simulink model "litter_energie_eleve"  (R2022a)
settings: Solver=ode14x  StartTime=0.0  StopTime=560  FixedStep=0.001  RelTol=1e-4  EnableMultiTasking=on
libraries: fl_lib x26, nesl_utility x12, ee_lib x2, simulink x1

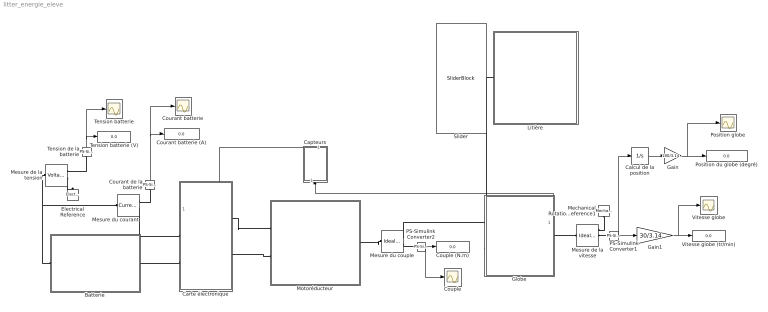
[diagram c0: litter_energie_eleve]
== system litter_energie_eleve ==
  Batterie : Subsystem
  Calcul de la position : Integrator
  Capteurs : Subsystem
  Carte électronique : Subsystem
  Couple : Scope
  Couple (N.m) : Display
  Courant batterie : Scope
  Courant batterie (A) : Display
  Courant de la batterie : nesl_utility/PS-Simulink Converter  PhysicalDomain=network_engine_domain  SubClassName=ps_output  LeftPortType=input  RightPortType=output  PseudoPeriodic=off  Frequencies=[]  VectorFormat=1-D array  Unit=inherit  AffineConversion=off
  Electrical Reference : fl_lib/Electrical/Electrical Elements/Electrical Reference
  Gain : Gain  Gain=180/3.14
  Gain1 : Gain  Gain=30/3.14
  Globe : Subsystem
  Litière : Subsystem
  Mechanical Rotational Reference1 : fl_lib/Mechanical/Rotational Elements/Mechanical Rotational Reference
  Mesure de la tension : fl_lib/Electrical/Electrical Sensors/Voltage Sensor
  Mesure de la vitesse : fl_lib/Mechanical/Mechanical Sensors/Ideal Rotational Motion Sensor  wrap_angle=simscape.enum.onoff.off  offset=0 rad
  Mesure du couple : fl_lib/Mechanical/Mechanical Sensors/Ideal Torque Sensor
  Mesure du courant : fl_lib/Electrical/Electrical Sensors/Current Sensor
  Motoréducteur : Subsystem
  PS-Simulink Converter1 : nesl_utility/PS-Simulink Converter  PhysicalDomain=network_engine_domain  SubClassName=ps_output  LeftPortType=input  RightPortType=output  PseudoPeriodic=off  Frequencies=[]  VectorFormat=1-D array  Unit=inherit  AffineConversion=off
  PS-Simulink Converter2 : nesl_utility/PS-Simulink Converter  PhysicalDomain=network_engine_domain  SubClassName=ps_output  LeftPortType=input  RightPortType=output  PseudoPeriodic=off  Frequencies=[]  VectorFormat=1-D array  Unit=inherit  AffineConversion=off
  Position du globe (degré) : Display
  Position globe : Scope
  Slider : SliderBlock  ScaleMax=4.5
  Tension batterie : Scope
  Tension batterie (V) : Display
  Tension de la batterie : nesl_utility/PS-Simulink Converter  PhysicalDomain=network_engine_domain  SubClassName=ps_output  LeftPortType=input  RightPortType=output  PseudoPeriodic=off  Frequencies=[]  VectorFormat=1-D array  Unit=inherit  AffineConversion=off
  Vitesse globe : Scope
  Vitesse globe (tr/min) : Display
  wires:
  Courant de la batterie/1 -> Courant batterie/1, Courant batterie (A)/1
  Tension de la batterie/1 -> Tension batterie/1, Tension batterie (V)/1
  Calcul de la position/1 -> Gain/1
  PS-Simulink Converter1/1 -> Calcul de la position/1, Gain1/1
  PS-Simulink Converter2/1 -> Couple/1, Couple (N.m)/1
  Globe/1(Out1) -> Capteurs/1(In1)
  Capteurs/1(Out1) -> Carte électronique/1(angle)
  Gain/1 -> Position globe/1, Position du globe (degré)/1
  Gain1/1 -> Vitesse globe/1, Vitesse globe (tr/min)/1
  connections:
  Courant de la batterie/LConn1 -- Mesure du courant/RConn1
  PS-Simulink Converter1/LConn1 -- Mesure de la vitesse/RConn2
  Mechanical Rotational Reference1/LConn1 -- Mesure de la vitesse/RConn1
  Tension de la batterie/LConn1 -- Mesure de la tension/RConn1
  Mesure de la tension/LConn1 -- Batterie/LConn1 -- Mesure du courant/LConn1
  Mesure de la tension/RConn2 -- Electrical Reference/LConn1
  Mesure du courant/RConn2 -- Carte électronique/LConn1
  Batterie/RConn1 -- Carte électronique/LConn2
  Carte électronique/RConn1 -- Motoréducteur/LConn1
  Carte électronique/RConn2 -- Motoréducteur/LConn2
  Mesure du couple/LConn1 -- Motoréducteur/RConn1
  Globe/RConn1 -- Mesure de la vitesse/LConn1
  Mesure du couple/RConn2 -- PS-Simulink Converter2/LConn1
  Mesure du couple/RConn1 -- Globe/LConn1
  Globe/LConn2 -- Litière/RConn1

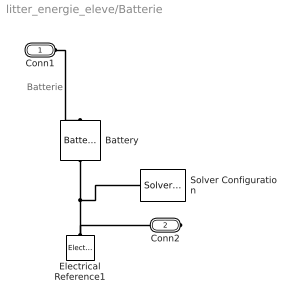
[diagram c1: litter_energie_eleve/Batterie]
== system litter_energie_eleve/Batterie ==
  note: Batterie
  Battery : ee_lib/Sources/Battery  Vnom=12 V  prm_dir=ee.enum.batterybasic.prm_dir.disabled  R1_dis=2 Ohm  R1_ch=2 Ohm  R1=2 Ohm  prm_AH=ee.enum.batterybasic.prm_AH.infinite  AH=50 A*hr  V1=11.5 V  AH1=25 A*hr  prm_R2=ee.enum.batterybasic.prm_R2.disabled  R2=2000 Ohm  prm_dyn=ee.enum.batterybasic.prm_dyn.off  Rp1=0.005 Ohm  tau1=30 s  Rp2=0.005 Ohm  tau2=30 s  Rp3=0.005 Ohm  tau3=30 s  Rp4=0.005 Ohm  tau4=30 s  Rp5=0.005 Ohm  tau5=30 s  prm_fade=ee.enum.batterybasic.prm_fade.disabled  N_fade=100  AH_fade=45 A*hr  R1_fade=2.02 Ohm  R1_ch_fade=2.02 Ohm  V1_fade=10.35 V  prm_age=ee.enum.batterybasic.prm_age.disabled  prm_age_OCV=ee.enum.batterybasic.prm_age_OCV.OCV  OCV_age=0.9  SOC_age=60  delta_time_age_vec=[0] d  temperature_age_vec=[273] K  OCV_scaling_age=2.2134e6  OCV_offset_age=1.632e6  temp_exp_age=0.515833569 V  t_exp_age=0.75  i_specify=off  i_priority=None  i=0 A  i_nominal_specify=off  i_nominal_unit=A  i_nominal_value=1  v_specify=off  v_priority=None  v=0 V  v_nominal_specify=off  v_nominal_unit=V  v_nominal_value=1  charge_specify=on  charge_priority=High  charge=13 A*hr  charge_nominal_specify=off  charge_nominal_unit=A*hr  charge_nominal_value=1  num_cycles_specify=off  num_cycles_priority=High  num_cycles=0  num_cycles_nominal_specify=off  num_cycles_nominal_unit=1  num_cycles_nominal_value=1  Tmeas=298.15 K  Tmeas_age=298.15 K  Vnom_T2=12 V  R1_T2=2.2 Ohm  R1_T2_dis=2.2 Ohm  R1_T2_ch=2.2 Ohm  V1_T2=11.4 V  R2_T2=2200 Ohm  Rp1_T2=0.005 Ohm  tau1_T2=30 s  Rp2_T2=0.005 Ohm  tau2_T2=30 s  Rp3_T2=0.005 Ohm  tau3_T2=30 s  Rp4_T2=0.005 Ohm  tau4_T2=30 s  Rp5_T2=0.005 Ohm  tau5_T2=30 s  Tmeas2=273.15 K  thermal_mass=30000 J/K  temperature_specify=off  temperature_priority=High  temperature=298.15 K  temperature_nominal_specify=off  temperature_nominal_unit=K  temperature_nominal_value=1
  Electrical Reference1 : fl_lib/Electrical/Electrical Elements/Electrical Reference
  Solver Configuration : nesl_utility/Solver Configuration  PhysicalDomain=network_engine_domain  SubClassName=solver  LeftPortType=input  RightPortType=generic  Tones=[]  Harmonics=[]  SimulateNoise=off  Profile=off  UseLocalSampling=off  EnableSwitchedLinearOptims=on  FrequencyDomain=off  UseCCode=off  RelTol=0.001  AbsTol=1e-06  MinStep=1e-09  ToWorkspace=off  RevertToSquareIcSolve=off  NumHomotopyIterations=100  PhasorMode=off  PhasorModeNumHarmonics=1  IndexReductionMethod=DerivativeReplacement  DoDC=off  ResidualTolerance=1e-4  UseLocalSolver=on  LocalSolverChoice=NE_TRAPEZOIDAL_ADVANCER  LocalSolverSampleTime=.001  DoFixedCost=on  MaxNonlinIter=3  MaxModeIter=2  ComputeImpulses=off  ImpulseIterations=2  LinearAlgebra=Sparse  LinearAlgebraNumThread=0  EquationFormulation=NE_TIME_EF  DelaysMemoryBudget=4096  AutomaticFiltering=on  FilteringTimeConstant=0.001  PartitionStorageMethod=AS_NEEDED  PartitionMemoryBudget=1024  PartitionMethod=FAST
  Conn1 : PMIOPort  Side=Left
  Conn2 : PMIOPort  Port=2  Side=Right
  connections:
  Electrical Reference1/LConn1 -- Conn2/RConn1 -- Battery/RConn1 -- Solver Configuration/RConn1
  Conn1/RConn1 -- Battery/LConn1

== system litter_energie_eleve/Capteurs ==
  In1 : Inport
  Integrator : Integrator
  Out1 : Outport
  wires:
  Integrator/1 -> Out1/1
  In1/1 -> Integrator/1

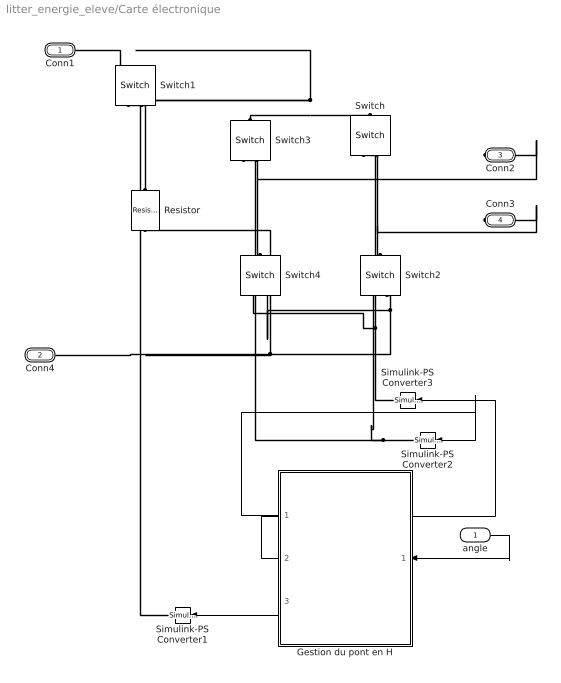
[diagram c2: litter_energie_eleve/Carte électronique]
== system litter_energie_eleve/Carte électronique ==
  angle : Inport
  Gestion du pont en H : Stateflow chart  TreatAsAtomicUnit=on
  Resistor : fl_lib/Electrical/Electrical Elements/Resistor  R=150 Ohm  i_specify=off  i_priority=None  i=0 A  i_nominal_specify=off  i_nominal_unit=A  i_nominal_value=1  v_specify=off  v_priority=None  v=0 V  v_nominal_specify=off  v_nominal_unit=V  v_nominal_value=1
  Simulink-PS Converter1 : nesl_utility/Simulink-PS Converter  PhysicalDomain=network_engine_domain  SubClassName=ps_input  LeftPortType=input  RightPortType=output  PseudoPeriodic=off  Frequencies=[]  NoiseDistribution=none  NoiseParameters=[]  Unit=1  AffineConversion=off  FilteringAndDerivatives=provide  SimscapeFilterOrder=1  InputFilterTimeConstant=0.001  UdotUserProvided=0
  Simulink-PS Converter2 : nesl_utility/Simulink-PS Converter  PhysicalDomain=network_engine_domain  SubClassName=ps_input  LeftPortType=input  RightPortType=output  PseudoPeriodic=off  Frequencies=[]  NoiseDistribution=none  NoiseParameters=[]  Unit=1  AffineConversion=off  FilteringAndDerivatives=provide  SimscapeFilterOrder=1  InputFilterTimeConstant=0.001  UdotUserProvided=0
  Simulink-PS Converter3 : nesl_utility/Simulink-PS Converter  PhysicalDomain=network_engine_domain  SubClassName=ps_input  LeftPortType=input  RightPortType=output  PseudoPeriodic=off  Frequencies=[]  NoiseDistribution=none  NoiseParameters=[]  Unit=1  AffineConversion=off  FilteringAndDerivatives=provide  SimscapeFilterOrder=1  InputFilterTimeConstant=0.001  UdotUserProvided=0
  Switch{,1..4} (5 alike) : fl_lib/Electrical/Electrical Elements/Switch  R_closed=0.01 Ohm  G_open=1e-8 1/Ohm  Threshold=0.5  i_specify=off  i_priority=None  i=0 A  i_nominal_specify=off  i_nominal_unit=A  i_nominal_value=1  v_specify=off  v_priority=None  v=0 V  v_nominal_specify=off  v_nominal_unit=V  v_nominal_value=1
  Conn1 : PMIOPort  Side=Left
  Conn4 : PMIOPort  Port=2  Side=Left
  Conn2 : PMIOPort  Port=3  Side=Right
  Conn3 : PMIOPort  Port=4  Side=Right
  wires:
  Gestion du pont en H/2(sens_neg) -> Simulink-PS Converter3/1
  angle/1 -> Gestion du pont en H/1(angle)
  Gestion du pont en H/1(sens_pos) -> Simulink-PS Converter2/1
  Gestion du pont en H/3(marche) -> Simulink-PS Converter1/1
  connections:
  Switch/RConn2 -- Conn3/RConn1 -- Switch2/LConn1
  Switch3/LConn1 -- Switch1/LConn1 -- Conn1/RConn1 -- Switch/LConn1
  Simulink-PS Converter2/RConn1 -- Switch2/RConn1 -- Switch3/RConn1
  Simulink-PS Converter3/RConn1 -- Switch4/RConn1 -- Switch/RConn1
  Switch2/RConn2 -- Resistor/RConn1 -- Conn4/RConn1 -- Switch4/RConn2
  Switch3/RConn2 -- Conn2/RConn1 -- Switch4/LConn1
  Resistor/LConn1 -- Switch1/RConn2
  Simulink-PS Converter1/RConn1 -- Switch1/RConn1

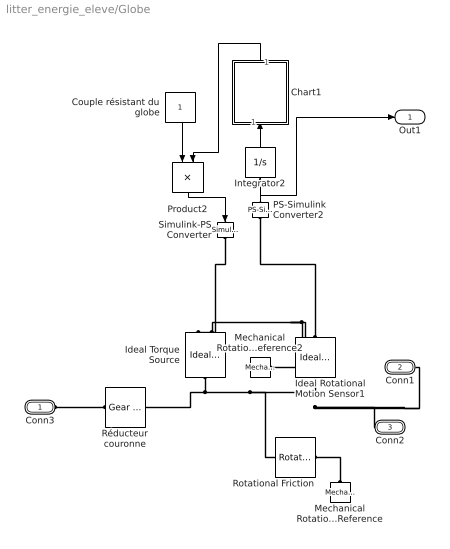
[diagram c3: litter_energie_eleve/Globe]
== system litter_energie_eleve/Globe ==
  Chart1 : Stateflow chart  TreatAsAtomicUnit=on
  Couple résistant du globe : Constant
  Ideal Rotational Motion Sensor1 : fl_lib/Mechanical/Mechanical Sensors/Ideal Rotational Motion Sensor  wrap_angle=simscape.enum.onoff.off  offset=0 rad
  Ideal Torque Source : fl_lib/Mechanical/Mechanical Sources/Ideal Torque Source
  Integrator2 : Integrator
  Mechanical Rotational Reference : fl_lib/Mechanical/Rotational Elements/Mechanical Rotational Reference
  Mechanical Rotational Reference2 : fl_lib/Mechanical/Rotational Elements/Mechanical Rotational Reference
  PS-Simulink Converter2 : nesl_utility/PS-Simulink Converter  PhysicalDomain=network_engine_domain  SubClassName=ps_output  LeftPortType=input  RightPortType=output  PseudoPeriodic=off  Frequencies=[]  VectorFormat=1-D array  Unit=inherit  AffineConversion=off
  Product2 : Product
  Rotational Friction : fl_lib/Mechanical/Rotational Elements/Rotational Friction  brkwy_trq=15 N*m  brkwy_vel=0.01 rad/s  Col_trq=9 N*m  visc_coef=0.0001 N*m*s/rad  w_specify=off  w_priority=None  w=0 rad/s  w_nominal_specify=off  w_nominal_unit=rad/s  w_nominal_value=1  t_specify=off  t_priority=None  t=0 N*m  t_nominal_specify=off  t_nominal_unit=N*m  t_nominal_value=1
  Réducteur couronne : fl_lib/Mechanical/Mechanisms/Gear Box  ratio=76/9  t_in_specify=off  t_in_priority=None  t_in=0 N*m  t_in_nominal_specify=off  t_in_nominal_unit=N*m  t_in_nominal_value=1  t_out_specify=off  t_out_priority=None  t_out=0 N*m  t_out_nominal_specify=off  t_out_nominal_unit=N*m  t_out_nominal_value=1
  Simulink-PS Converter : nesl_utility/Simulink-PS Converter  PhysicalDomain=network_engine_domain  SubClassName=ps_input  LeftPortType=input  RightPortType=output  PseudoPeriodic=off  Frequencies=[]  NoiseDistribution=none  NoiseParameters=[]  Unit=N*m  AffineConversion=off  FilteringAndDerivatives=provide  SimscapeFilterOrder=1  InputFilterTimeConstant=0.001  UdotUserProvided=0
  Conn3 : PMIOPort  Side=Left
  Conn1 : PMIOPort  Port=2  Side=Left
  Conn2 : PMIOPort  Port=3  Side=Right
  Out1 : Outport
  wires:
  Couple résistant du globe/1 -> Product2/1
  Product2/1 -> Simulink-PS Converter/1
  PS-Simulink Converter2/1 -> Out1/1, Integrator2/1
  Chart1/1(signe_couple_LR) -> Product2/2
  Integrator2/1 -> Chart1/1(angle)
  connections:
  Ideal Torque Source/RConn2 -- Ideal Rotational Motion Sensor1/RConn1 -- Mechanical Rotational Reference2/LConn1
  Simulink-PS Converter/RConn1 -- Ideal Torque Source/RConn1
  Ideal Torque Source/LConn1 -- Réducteur couronne/RConn1 -- Rotational Friction/LConn1 -- Conn1/RConn1 -- Conn2/RConn1 -- Ideal Rotational Motion Sensor1/LConn1
  PS-Simulink Converter2/LConn1 -- Ideal Rotational Motion Sensor1/RConn2
  Réducteur couronne/LConn1 -- Conn3/RConn1
  Mechanical Rotational Reference/LConn1 -- Rotational Friction/RConn1

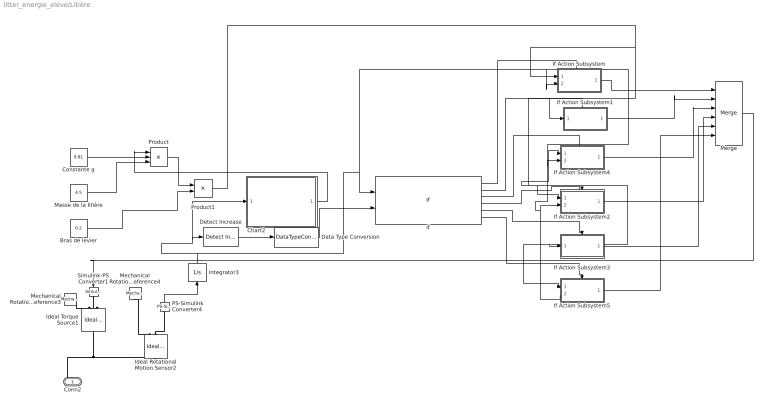
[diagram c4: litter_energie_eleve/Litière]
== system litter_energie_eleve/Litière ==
  Bras de levier : Constant  Value=0.2
  Chart2 : Stateflow chart  TreatAsAtomicUnit=on
  Constante g : Constant  Value=9.81
  Data Type Conversion : DataTypeConversion
  Detect Increase : simulink/Logic and Bit Operations/Detect Increase  vinit=0.0  OutDataTypeStr=boolean
  Ideal Rotational Motion Sensor2 : fl_lib/Mechanical/Mechanical Sensors/Ideal Rotational Motion Sensor  wrap_angle=simscape.enum.onoff.off  offset=0 rad
  Ideal Torque Source1 : fl_lib/Mechanical/Mechanical Sources/Ideal Torque Source
  If : If  NumInputs=2  IfExpression=(u1>=0)&(u1 < 0.785) & (u2 == 1)  ElseIfExpressions=(u1 >= 0.785) & (u2 == 1),(u1>3.14)&(u2==0), (u1>2.36)&(u2==0),(u1>-0.785) & (u2 == 0), (u1<0)&(u2 == 1)  ShowElse=off
  If Action Subsystem : Subsystem  TreatAsAtomicUnit=on
  If Action Subsystem1 : Subsystem  TreatAsAtomicUnit=on
  If Action Subsystem2 : Subsystem  TreatAsAtomicUnit=on
  If Action Subsystem3 : Subsystem  TreatAsAtomicUnit=on
  If Action Subsystem4 : Subsystem  TreatAsAtomicUnit=on
  If Action Subsystem5 : Subsystem  TreatAsAtomicUnit=on
  Integrator3 : Integrator
  Masse de la litière : Constant  Value=4.5
  Mechanical Rotational Reference3 : fl_lib/Mechanical/Rotational Elements/Mechanical Rotational Reference
  Mechanical Rotational Reference4 : fl_lib/Mechanical/Rotational Elements/Mechanical Rotational Reference
  Merge : Merge  Inputs=6
  PS-Simulink Converter4 : nesl_utility/PS-Simulink Converter  PhysicalDomain=network_engine_domain  SubClassName=ps_output  LeftPortType=input  RightPortType=output  PseudoPeriodic=off  Frequencies=[]  VectorFormat=1-D array  Unit=inherit  AffineConversion=off
  Product : Product  Inputs=3
  Product1 : Product
  Simulink-PS Converter1 : nesl_utility/Simulink-PS Converter  PhysicalDomain=network_engine_domain  SubClassName=ps_input  LeftPortType=input  RightPortType=output  PseudoPeriodic=off  Frequencies=[]  NoiseDistribution=none  NoiseParameters=[]  Unit=1  AffineConversion=off  FilteringAndDerivatives=provide  SimscapeFilterOrder=1  InputFilterTimeConstant=0.001  UdotUserProvided=0
  Conn2 : PMIOPort  Side=Right
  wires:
  If/5 -> If Action Subsystem3/Action
  If/3 -> If Action Subsystem4/Action
  Integrator3/1 -> Detect Increase/1, Chart2/1(angle), If Action Subsystem4/2(In2), If Action Subsystem2/2(In3), If Action Subsystem5/2(In3), If Action Subsystem/2(In1), If/1
  If/4 -> If Action Subsystem2/Action
  If Action Subsystem5/1(Out1) -> Merge/6
  If/6 -> If Action Subsystem5/Action
  If Action Subsystem3/1(Out1) -> Merge/5
  Masse de la litière/1 -> Product/3
  If Action Subsystem1/1(Out1) -> Merge/2
  If Action Subsystem2/1(Out1) -> Merge/4
  If Action Subsystem4/1(Out1) -> Merge/3
  Product/1 -> Product1/1
  Chart2/1(signe_couple_litiere) -> Product/1
  Merge/1 -> Simulink-PS Converter1/1
  Product1/1 -> If Action Subsystem5/1(In1), If Action Subsystem3/1(In1), If Action Subsystem2/1(In1), If Action Subsystem4/1(In1), If Action Subsystem1/1(In1), If Action Subsystem/1(In2)
  PS-Simulink Converter4/1 -> Integrator3/1
  Bras de levier/1 -> Product1/2
  Detect Increase/1 -> Data Type Conversion/1
  If/2 -> If Action Subsystem1/Action
  Data Type Conversion/1 -> If/2
  If/1 -> If Action Subsystem/Action
  If Action Subsystem/1(Out1) -> Merge/1
  Constante g/1 -> Product/2
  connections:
  Ideal Rotational Motion Sensor2/LConn1 -- Conn2/RConn1 -- Ideal Torque Source1/LConn1
  Mechanical Rotational Reference3/LConn1 -- Ideal Torque Source1/RConn2
  Ideal Rotational Motion Sensor2/RConn2 -- PS-Simulink Converter4/LConn1
  Ideal Rotational Motion Sensor2/RConn1 -- Mechanical Rotational Reference4/LConn1
  Simulink-PS Converter1/RConn1 -- Ideal Torque Source1/RConn1

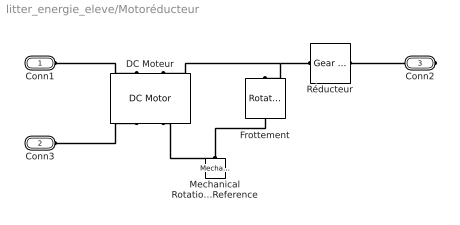
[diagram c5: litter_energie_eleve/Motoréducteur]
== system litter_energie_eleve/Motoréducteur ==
  DC Moteur : ee_lib/Electromechanical/Brushed Motors/DC Motor  field_option=ee.enum.field_option.pm  Rf=100 Ohm  Lf=1 H  Laf=0.15 H  If0=0 A  parameterization=ee.enum.dcparam_option.circuit_param  Ra=9 Ohm  La=4.5 mH  emf_or_torque=ee.enum.emf_or_torque.kv  Kv=0.016 V/(rad/s)  Ki=0.0001 N*m/A  T_stall=0.059 N*m  w_max=7300 rpm  w_rated=6636 rpm  P_rated=1.31 W  V_rated=12 V  lam_param=ee.enum.lam_param.current  i_noload=0.15 A  V_i_noload=100 V  J=0.00001 kg*m^2  lam=0 N*m/(rad/s)  speed0=0 rpm  enable_fault_armature=simscape.enum.onoff.off  rev_faulted=1 / 3  G_faulted_armature=1e-5 S  fault_trigger_armature=ee.enum.faults.faultTrigger.temporal  t_fault_armature=1 s  max_permissible_current_armature=inf A  t_fail_on_current_armature=1 s  enable_fault_field=simscape.enum.onoff.off  G_faulted_field=1e-5 S  fault_trigger_field=ee.enum.faults.faultTrigger.temporal  t_fault_field=1 s  max_permissible_current_field=inf A  t_fail_on_current_field=1 s  fault_action=simscape.enum.assert.action.none  alpha=3.93e-3 1/K  Tmeas=25 degC  thermal_mass=100 J/K  initial_temperature=25 degC
  Frottement : fl_lib/Mechanical/Rotational Elements/Rotational Friction  brkwy_trq=0.00008 N*m  brkwy_vel=0.060623 rad/s  Col_trq=0.000072 N*m  visc_coef=0.68e-6 N*m*s/rad  w_specify=off  w_priority=None  w=0 rad/s  w_nominal_specify=off  w_nominal_unit=rad/s  w_nominal_value=1  t_specify=off  t_priority=None  t=0 N*m  t_nominal_specify=off  t_nominal_unit=N*m  t_nominal_value=1
  Mechanical Rotational Reference : fl_lib/Mechanical/Rotational Elements/Mechanical Rotational Reference
  Réducteur : fl_lib/Mechanical/Mechanisms/Gear Box  ratio=1420  t_in_specify=off  t_in_priority=None  t_in=0 N*m  t_in_nominal_specify=off  t_in_nominal_unit=N*m  t_in_nominal_value=1  t_out_specify=off  t_out_priority=None  t_out=0 N*m  t_out_nominal_specify=off  t_out_nominal_unit=N*m  t_out_nominal_value=1
  Conn1 : PMIOPort  Side=Left
  Conn3 : PMIOPort  Port=2  Side=Left
  Conn2 : PMIOPort  Port=3  Side=Right
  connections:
  Conn3/RConn1 -- DC Moteur/RConn1
  Mechanical Rotational Reference/LConn1 -- DC Moteur/RConn2 -- Frottement/RConn1
  Réducteur/LConn1 -- DC Moteur/LConn2 -- Frottement/LConn1
  Conn2/RConn1 -- Réducteur/RConn1
  Conn1/RConn1 -- DC Moteur/LConn1

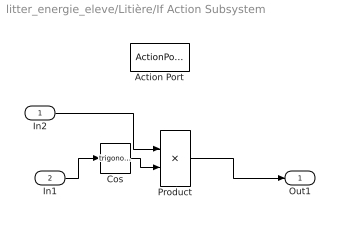
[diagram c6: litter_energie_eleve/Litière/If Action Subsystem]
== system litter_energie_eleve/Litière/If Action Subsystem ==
  In2 : Inport
  In1 : Inport  Port=2
  Action Port : ActionPort  ActionPortLabel=if((u1>=0)&(u1 < 0.785) & (u2 == 1))
  Cos : Trigonometry
  Product : Product
  Out1 : Outport
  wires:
  Product/1 -> Out1/1
  In2/1 -> Product/1
  Cos/1 -> Product/2
  In1/1 -> Cos/1

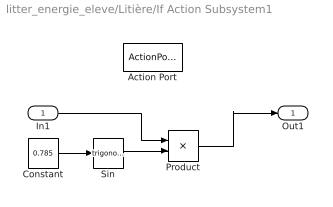
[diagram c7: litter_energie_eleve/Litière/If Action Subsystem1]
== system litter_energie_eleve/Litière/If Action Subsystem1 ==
  In1 : Inport
  Action Port : ActionPort  ActionPortLabel=elseif((u1 >= 0.785) & (u2 == 1))
  Constant : Constant  Value=0.785
  Product : Product
  Sin : Trigonometry
  Out1 : Outport
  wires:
  Sin/1 -> Product/2
  In1/1 -> Product/1
  Constant/1 -> Sin/1
  Product/1 -> Out1/1

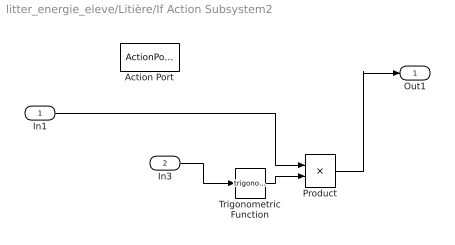
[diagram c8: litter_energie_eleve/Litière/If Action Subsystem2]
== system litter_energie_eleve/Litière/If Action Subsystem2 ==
  In1 : Inport
  In3 : Inport  Port=2
  Action Port : ActionPort  ActionPortLabel=elseif( (u1>2.36)&(u2==0))
  Product : Product
  Trigonometric Function : Trigonometry
  Out1 : Outport
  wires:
  Trigonometric Function/1 -> Product/2
  In3/1 -> Trigonometric Function/1
  In1/1 -> Product/1
  Product/1 -> Out1/1

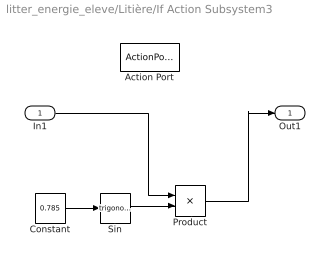
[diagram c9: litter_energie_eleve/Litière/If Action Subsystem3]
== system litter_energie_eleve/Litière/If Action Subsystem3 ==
  In1 : Inport
  Action Port : ActionPort  ActionPortLabel=elseif((u1>-0.785) & (u2 == 0))
  Constant : Constant  Value=0.785
  Product : Product
  Sin : Trigonometry
  Out1 : Outport
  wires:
  Constant/1 -> Sin/1
  Sin/1 -> Product/2
  In1/1 -> Product/1
  Product/1 -> Out1/1

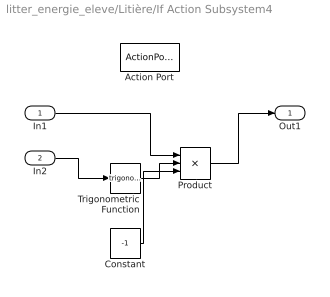
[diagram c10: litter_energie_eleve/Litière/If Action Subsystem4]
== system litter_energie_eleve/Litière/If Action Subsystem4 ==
  In1 : Inport
  In2 : Inport  Port=2
  Action Port : ActionPort  ActionPortLabel=elseif((u1>3.14)&(u2==0))
  Constant : Constant  Value=-1
  Product : Product  Inputs=3
  Trigonometric Function : Trigonometry
  Out1 : Outport
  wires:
  Constant/1 -> Product/3
  In1/1 -> Product/1
  Trigonometric Function/1 -> Product/2
  In2/1 -> Trigonometric Function/1
  Product/1 -> Out1/1

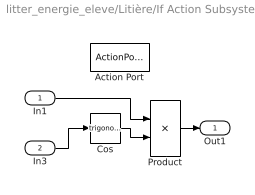
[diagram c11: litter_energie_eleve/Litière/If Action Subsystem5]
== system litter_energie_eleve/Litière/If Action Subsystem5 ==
  In1 : Inport
  In3 : Inport  Port=2
  Action Port : ActionPort  ActionPortLabel=elseif( (u1<0)&(u2 == 1))
  Cos : Trigonometry
  Product : Product
  Out1 : Outport
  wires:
  Product/1 -> Out1/1
  In3/1 -> Cos/1
  Cos/1 -> Product/2
  In1/1 -> Product/1

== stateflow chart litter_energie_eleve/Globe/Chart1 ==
  state Rotation_anti_horaire1
    entry: signe_couple_LR = -1;
  state Rotation_horaire
    entry: signe_couple_LR = 1;
  state Rotation_anti_horaire2
    entry: signe_couple_LR = -1;
  state Arret
    entry: signe_couple_LR = 0;
  (default) -> Rotation_anti_horaire1
  Rotation_anti_horaire1 -> Rotation_horaire : [angle>3.93]
  Rotation_horaire -> Rotation_anti_horaire2 : [angle<-0.785]
  Rotation_anti_horaire2 -> Arret : [angle >0.1]
  data: angle input; signe_couple_LR output

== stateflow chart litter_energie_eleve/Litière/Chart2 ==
  state Tamisage
    entry: signe_couple_litiere = -1;
  state Couple_non_resistant
    entry: signe_couple_litiere=-1;
  state Retour
    entry: signe_couple_litiere=+1;
  state Retour1_position_initiale
    entry: signe_couple_litiere = -1;
  state Arret
    entry: signe_couple_litiere = 0;
  (default) -> Tamisage
  Tamisage -> Couple_non_resistant : [angle>3.93]
  Couple_non_resistant -> Retour : [angle<3.14]
  Retour -> Retour1_position_initiale : [angle<-0.785]
  Retour1_position_initiale -> Arret : [angle>0]
  data: angle input; signe_couple_litiere output

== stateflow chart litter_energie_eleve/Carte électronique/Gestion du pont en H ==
  state Attente_chat
    entry: marche = 0;
    sens_pos = 0;
    sens_neg = 0;
  state Detection_chat_et_attente
    entry: marche = 1;
    sens_pos = 0;
    sens_neg = 0;
  state Tamisage
    entry: sens_pos = 1;
    sens_neg = 0;
  state Pause
    entry: sens_pos = 0;
    sens_neg = 0;
  state Couple_non_resistant
    entry: sens_pos = 0;
    sens_neg = 1;
  state Retour
    entry: sens_pos = 0;
    sens_neg = 1;
  state Retour1_position_initiale
    entry: sens_pos = 1;
    sens_neg = 0;
  state Arret_moteur
    entry: sens_pos = 0;
    sens_neg = 0;
  state Mise_en_veille
    entry: marche = 0;
  (default) -> Attente_chat
  Attente_chat -> Detection_chat_et_attente : [after(10, sec)]
  Detection_chat_et_attente -> Tamisage : [after(180,sec)]
  Tamisage -> Pause : [angle>3.93]
  Pause -> Couple_non_resistant : after(2,sec)
  Couple_non_resistant -> Retour : [angle<3.14]
  Retour -> Retour1_position_initiale : [angle<-0.785]
  Retour1_position_initiale -> Arret_moteur : [angle>0]
  Arret_moteur -> Mise_en_veille : [after(180,sec)]
  data: angle input; sens_pos output; sens_neg output; marche output
